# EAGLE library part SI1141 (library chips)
AMBIENT LIGHT SENSOR
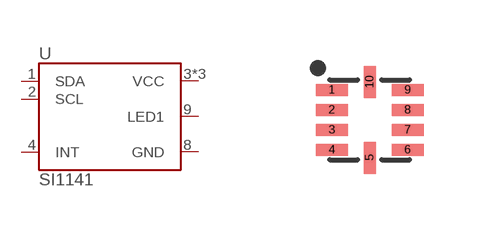
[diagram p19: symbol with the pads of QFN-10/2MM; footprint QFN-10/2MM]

Designator prefix U

## SI1141 (DIGIKEY: 336-2199-1-ND)  [QFN-10/2MM]
1  SDA
2  SCL
3  VCC
4  INT
6  VCC
7  VCC
8  GND
9  LED1

## Footprint QFN-10/2MM (pad centres in mm)
smd 0.8 x 0.3: 1 -0.95,0.75; 2 -0.95,0.25; 3 -0.95,-0.25; 4 -0.95,-0.75; 6 0.95,-0.75; 7 0.95,-0.25; 8 0.95,0.25; 9 0.95,0.75
smd 0.3 x 0.8: 5 0,-0.95; 10 0,0.95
